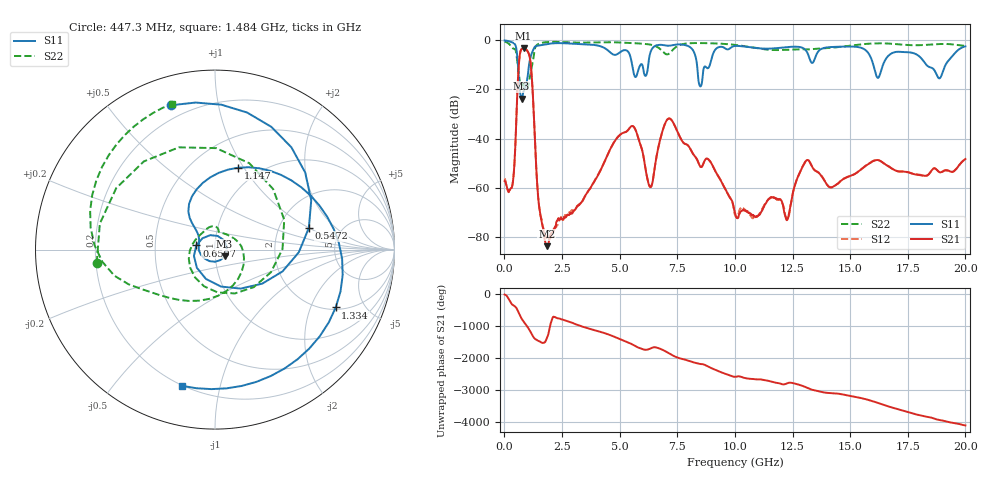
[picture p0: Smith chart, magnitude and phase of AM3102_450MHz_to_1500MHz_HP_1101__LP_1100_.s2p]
!Agilent Technologies,E8364B,MY43040894,A.07.50.67
!Agilent E8364B: A.07.50.67
!Date: Thursday, January 11, 2018 06:40:30
!Correction: S11(Full 2 Port(1,2))
!S21(Full 2 Port(1,2))
!S12(Full 2 Port(1,2))
!S22(Full 2 Port(1,2))
!S2P File: Measurements: S11, S21, S12, S22:
# Hz S  dB  R 50
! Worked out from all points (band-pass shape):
!   1601 points, 10 MHz to 20 GHz, reference 50 ohm
!   highest |S21| = -3.28 dB at 834.6 MHz (marker M1); lowest = -83.8 dB at 1.834 GHz (marker M2)
!   |S21| within 3 dB of the highest: 663.8 MHz to 1.084 GHz (420.6 MHz wide, 48.1 % of centre)
!   lowest |S11| = -23.7 dB at 747.1 MHz (marker M3), VSWR 1.14, Z = 55.4 - j4.2 ohm
!   |S11| at or under -10 dB: 586.1 MHz to 1.069 GHz (482.8 MHz wide, 58.3 % of centre); 8.357 GHz to 8.915 GHz (557.7 MHz wide, 6.46 % of centre); 18.31 GHz to 19.14 GHz (829.9 MHz wide, 4.43 % of centre)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
!   |S22| runs from -20.0 to -0.5 dB; largest |S21 - S12| = 0.00078
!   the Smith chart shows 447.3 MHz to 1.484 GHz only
!   S11 on the Smith chart (normalised r, x): 447.3 MHz: 0.13, +0.73; 547.2 MHz: 2.94, +1.00; 659.7 MHz: 0.81, +0.04; 1.147 GHz: 0.80, +0.94; 1.334 GHz: 2.10, -3.05; 1.484 GHz: 0.20, -0.77
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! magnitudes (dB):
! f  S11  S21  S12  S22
! 10 MHz  -0.1  -57.3  -56.3  -0.5
! 447.3 MHz  -1.5  -48.3  -48.5  -3.6
! 547.2 MHz  -5.4  -24.5  -24.5  -7.5
! 659.7 MHz  -19.4  -6.6  -6.6  -16.2
! 747.1 MHz  -23.7  -3.6  -3.6  -18.4
! 834.6 MHz  -20.7  -3.3  -3.3  -17.9
! 1.147 GHz  -6.5  -10.2  -10.2  -13.0
! 1.334 GHz  -2.5  -42.4  -42.5  -3.1
! 1.484 GHz  -2.1  -65.7  -65.8  -1.4
! 1.834 GHz  -1.5  -83.8  -80.5  -0.8
! 3.346 GHz  -1.6  -66.0  -65.8  -0.9
! 5.482 GHz  -7.2  -35.2  -35.2  -1.1
! 6.319 GHz  -5.4  -59.7  -59.6  -1.7
! 6.682 GHz  -1.9  -43.5  -43.5  -3.0
! 7.219 GHz  -2.1  -32.1  -32.1  -4.8
! 8.493 GHz  -18.7  -51.3  -51.3  -1.1
! 10.01 GHz  -2.3  -70.2  -71.1  -1.9
! 12.27 GHz  -2.8  -73.1  -72.6  -3.9
! 13.34 GHz  -9.2  -51.3  -51.3  -3.6
! 16.68 GHz  -6.1  -51.4  -51.3  -1.3
! 18.88 GHz  -15.5  -53.7  -53.7  -1.5
! 20 GHz  -2.5  -48.3  -48.5  -2.3
